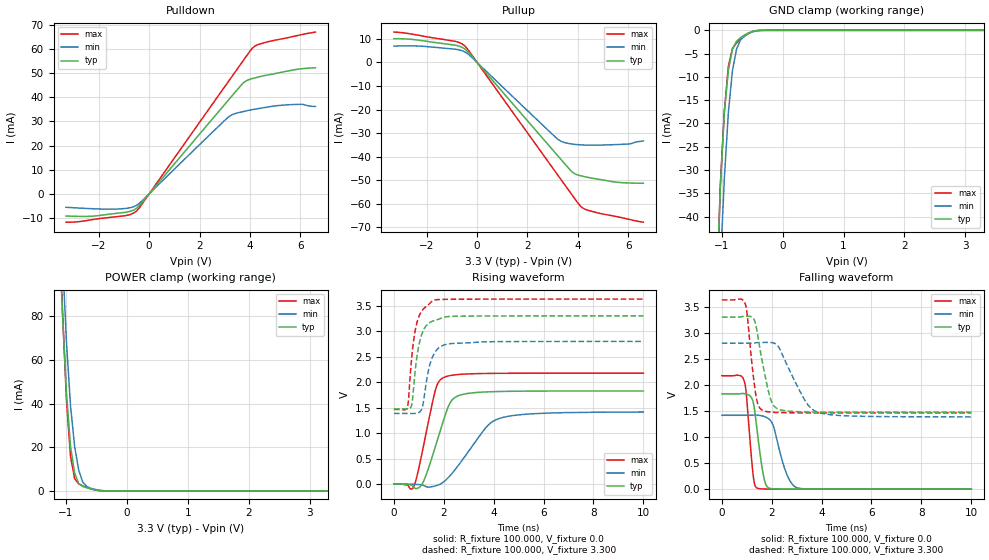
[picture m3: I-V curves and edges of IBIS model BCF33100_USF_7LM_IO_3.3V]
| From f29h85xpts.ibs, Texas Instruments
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|BCF33100_USF_7LM_IO_3.3V;
|   Model BCF33100_USF_7LM_IO_3.3V
[Model]   BCF33100_USF_7LM_IO_3.3V
Model_type   I/O
Polarity   Non-Inverting
Enable   Active-Low
Vinl =   0.800V
Vinh =   2.000V
Vmeas =  1.650V
Cref =   15.000pF
Vref =   0.0V
|   typ   min   max
C_comp   0.583pF   0.583pF   0.601pF
[Model Spec]
Vinh   2.000V   2.000V   2.000V
Vinl   0.800V   0.800V   0.800V
[Temperature Range]   25   155   -40
[Voltage Range]   3.300V   2.800V   3.630V
[Pullup Reference]   3.300V   2.800V   3.630V
[Pulldown Reference]   0.0V   0.0V   0.0V
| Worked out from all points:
|   slope of the pulldown table from 0 to 0.495 V, typ, clamps not added: 80.6 ohm
|   slope of the pullup table from 0 to 0.495 V, typ, clamps not added: 80.4 ohm
|   GND clamp passes 1 mA (typ) near -0.62 V on its own axis
|   POWER clamp passes 1 mA (typ) near -0.60 V on its own axis
|   rising waveform, R_fixture 100.000, V_fixture 0.0: 20-80 % time 711ps typ, 1.28ns min, 558ps max; typ from 0.002 V to 1.83 V
|   rising waveform, R_fixture 100.000, V_fixture 3.300: 20-80 % time 334ps typ, 367ps min, 321ps max; typ from 1.48 V to 3.3 V
|   falling waveform, R_fixture 100.000, V_fixture 0.0: 20-80 % time 301ps typ, 494ps min, 224ps max; typ from 1.83 V to 0.002 V
|   falling waveform, R_fixture 100.000, V_fixture 3.300: 20-80 % time 445ps typ, 893ps min, 286ps max; typ from 3.3 V to 1.48 V
[Pulldown]
|Voltage   I(typ)   I(min)   I(max)
-3.3V     -9.216mA   -5.594mA   -11.77mA
-2.1V     -9.148mA   -6.249mA   -10.45mA
-900mV    -7.597mA   -6.021mA   -8.98mA
-500mV    -6.002mA   -4.803mA   -7.149mA
3.1V      38.25mA    31.37mA    45.84mA
3.3V      40.71mA    32.81mA    48.79mA
3.7V      45.55mA    33.96mA    54.68mA
4.1V      47.75mA    34.88mA    60.36mA
4.4V      48.56mA    35.43mA    62.08mA
5.6V      51.06mA    36.92mA    64.9mA
6.1V      51.85mA    37.05mA    66.04mA
6.6V      52.19mA    36.16mA    66.99mA
[Pullup]
|Voltage   I(typ)   I(min)   I(max)
-3.3V     10.12mA    6.98mA     12.93mA
-2.3V     9.459mA    6.969mA    11.54mA
-900mV    7.427mA    5.697mA    9.065mA
-500mV    5.876mA    4.577mA    7.203mA
-200mV    2.513mA    2.07mA     3.035mA
3.2V      -39.63mA   -32.59mA   -47.84mA
3.4V      -42.1mA    -33.82mA   -50.82mA
3.8V      -46.79mA   -34.74mA   -56.78mA
4.1V      -48.15mA   -35.04mA   -61.06mA
4.5V      -49.08mA   -35.16mA   -63.17mA
6V        -51.25mA   -34.67mA   -66.64mA
6.6V      -51.37mA   -33.39mA   -67.93mA
[GND_clamp]
|Voltage   I(typ)   I(min)   I(max)
-3.3V     -1.438A    -1.047A    -2.083A
-1.089V   -60.71mA   -73.85mA   -63.17mA
-1.022V   -34.26mA   -51.29mA   -33.62mA
-955mV    -17.63mA   -31.99mA   -17.52mA
-888mV    -8.552mA   -17.56mA   -7.647mA
-821mV    -3.996mA   -8.625mA   -3.912mA
-754mV    -2.328mA   -4.033mA   -2.699mA
-687mV    -1.558mA   -2.027mA   -1.923mA
-620mV    -985.6uA   -1.136mA   -1.242mA
-553mV    -515.3uA   -630.1uA   -667.8uA
-352mV    -5.301uA   -28.14uA   -5.934uA
3.3V      0A         0A         0A
[POWER_clamp]
|Voltage   I(typ)   I(min)   I(max)
-3.3V     1.937A     2.196A     2.115A
-1.122V   126.5mA    155.3mA    134.7mA
-1.055V   81.92mA    108mA      83.97mA
-988mV    44.8mA     68.16mA    41.53mA
-921mV    20.34mA    38.89mA    15.71mA
-854mV    8.169mA    20.38mA    5.637mA
-787mV    3.403mA    9.476mA    3.185mA
-720mV    2.085mA    4.006mA    2.321mA
-653mV    1.432mA    1.972mA    1.599mA
-586mV    902uA      1.175mA    957.3uA
-318mV    6.47uA     41.69uA    3.141uA
3.3V      0A         0A         0A
[Ramp]
| variable   typ   min   max
dV/dt_r   1.095/0.711n   0.849/1.282n   1.304/0.558n
dV/dt_f   1.094/0.445n   0.848/0.892n   1.299/0.285n
R_load = 100.000
[Rising Waveform]
R_fixture= 100.000
V_fixture= 0.0
V_fixture_min= 0.0
V_fixture_max= 0.0
|time   V(typ)   V(min)   V(max)
0s        1.656mV    975.3uV    1.819mV
800ps     -62.84mV   -1.792mV   -40.96mV
1.166ns   35.83mV    -20.47mV   704.1mV
1.667ns   745.2mV    -33.25mV   1.85V
2.02ns    1.299V     56.08mV    2.097V
2.26ns    1.599V     172.8mV    2.13V
2.536ns   1.724V     338.9mV    2.148V
3.665ns   1.808V     1.096V     2.17V
4.245ns   1.817V     1.291V     2.173V
10ns      1.827V     1.415V     2.176V
[Rising Waveform]
R_fixture= 100.000
V_fixture= 3.300
V_fixture_min= 2.800
V_fixture_max= 3.630
|time   V(typ)   V(min)   V(max)
0s        1.476V     1.386V     1.463V
545ps     1.474V     1.387V     1.512V
703ps     1.536V     1.386V     2.431V
799ps     1.938V     1.386V     2.848V
931ps     2.526V     1.394V     3.179V
1.091ns   2.9V       1.448V     3.375V
1.395ns   3.154V     2.251V     3.524V
1.575ns   3.201V     2.524V     3.599V
2.445ns   3.292V     2.761V     3.625V
10ns      3.299V     2.799V     3.629V
[Falling Waveform]
R_fixture= 100.000
V_fixture= 0.0
V_fixture_min= 0.0
V_fixture_max= 0.0
|time   V(typ)   V(min)   V(max)
0s        1.827V     1.417V     2.176V
890ps     1.833V     1.417V     2.085V
979ps     1.825V     1.417V     1.832V
1.253ns   1.675V     1.42V      278.6mV
1.41ns    1.144V     1.421V     23.14mV
1.787ns   66.73mV    1.377V     4.192mV
2.061ns   8.447mV    1.219V     3.189mV
2.619ns   3.325mV    271.1mV    2.41mV
3.046ns   2.623mV    23.09mV    2.124mV
10ns      1.649mV    1.05mV     1.808mV
[Falling Waveform]
R_fixture= 100.000
V_fixture= 3.300
V_fixture_min= 2.800
V_fixture_max= 3.630
|time   V(typ)   V(min)   V(max)
0s        3.299V     2.799V     3.629V
934ps     3.314V     2.799V     3.558V
1.014ns   3.315V     2.799V     3.359V
1.368ns   3.141V     2.808V     1.793V
1.677ns   2.308V     2.813V     1.504V
1.951ns   1.733V     2.814V     1.479V
2.151ns   1.567V     2.787V     1.472V
3.364ns   1.482V     1.678V     1.464V
3.824ns   1.479V     1.482V     1.464V
10ns      1.476V     1.387V     1.463V
